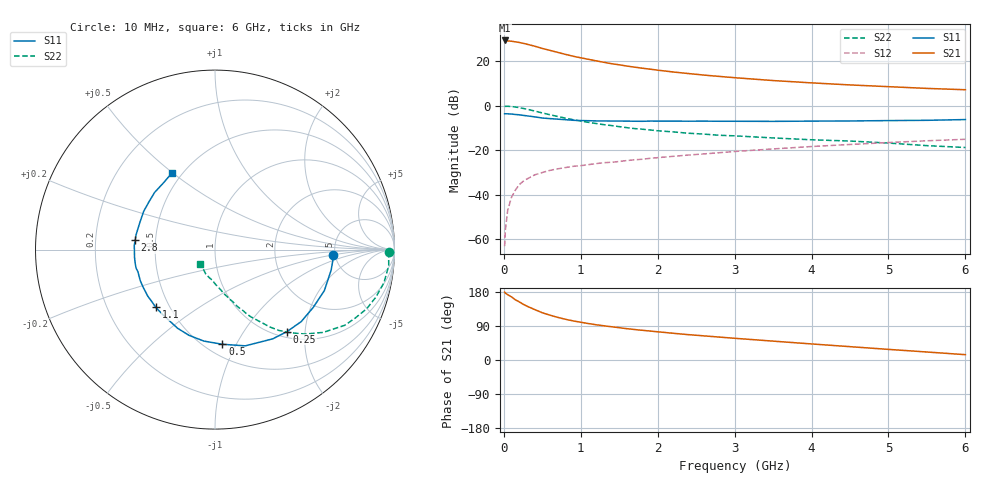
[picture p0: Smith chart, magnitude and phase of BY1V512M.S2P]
! SIEMENS Small Signal Semiconductors
! BFY420
! Si NPN RF SIEGET Grounded Emitter Transistor in MICRO-X
! VCE = 1.5 V  IC = 12 mA
! Common Emitter S-Parameters:  October  1996
# GHz  S  MA  R  50
!  f  S11  S21  S12  S22
! GHz  MAG  ANG  MAG  ANG  MAG  ANG  MAG  ANG
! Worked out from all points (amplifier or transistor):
!   36 points, 10 MHz to 6 GHz, reference 50 ohm
!   highest |S21| = 29.3 dB at 10 MHz (marker M1)
!   |S21| within 3 dB of that: start of sweep to 442.8 MHz
!   unconditionally stable (mu >= 1): 2.306 GHz to end of sweep
!   at 250 MHz: K = 0.22, MSG = 31.0 dB, |S12| = -34.0 dB
!   at 1.4 GHz: K = 0.81, MSG = 22.1 dB, |S12| = -25.4 dB
!   at 6 GHz: K = 1.10, MAG = 9.2 dB, |S12| = -15.1 dB
!   S11 on the Smith chart (normalised r, x): 10 MHz: 4.82, -0.47; 250 MHz: 1.11, -1.61; 500 MHz: 0.60, -0.88; 1.1 GHz: 0.42, -0.34; 2.8 GHz: 0.38, +0.05; 6 GHz: 0.44, +0.49
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0.01  0.6591 -2.4  29.24 179.1  0.0007 86.8  0.9713 -0.8
0.02  0.6601 -4.5  29.21 176.4  0.0016 86.1  0.968 -1.9
0.05  0.6572 -10.0  28.47 172.4  0.0045 81.5  0.9722 -5.3
0.1  0.6507 -20.6  28.13 166.5  0.0088 81.4  0.9592 -11.1
0.15  0.6351 -30.4  27.21 158.9  0.0127 75.8  0.9349 -16.4
0.2  0.6258 -39.9  26.41 153.5  0.0168 72.6  0.9073 -21.3
0.25  0.608 -48.7  25.27 147.3  0.02 68.2  0.8703 -25.9
0.3  0.5922 -57.1  24.07 142.1  0.0226 65.6  0.8375 -30.2
0.4  0.5622 -72.5  21.77 133.2  0.0279 61.0  0.7593 -37.4
0.5  0.5292 -85.5  19.35 124.7  0.0316 57.2  0.6886 -43.1
0.6  0.5134 -97.0  17.47 118.3  0.0353 54.2  0.6266 -47.7
0.8  0.4854 -115.4  14.24 107.5  0.0408 50.5  0.5264 -54.8
0.9  0.4709 -122.6  12.94 103.2  0.0435 50.1  0.4853 -57.2
1.1  0.4608 -135.7  11.03 96.1  0.0475 49.8  0.4235 -62.0
1.3  0.4556 -145.2  9.449 90.3  0.0525 49.1  0.3754 -65.2
1.6  0.4509 -157.6  7.766 82.6  0.0587 48.9  0.3214 -70.0
2.2  0.4505 -174.4  5.727 70.6  0.073 48.0  0.2583 -77.3
2.8  0.4477 173.3  4.552 60.5  0.0879 46.0  0.2168 -83.6
3.5  0.4451 160.3  3.675 49.8  0.107 42.4  0.189 -90.3
4.5  0.4543 144.0  2.931 35.2  0.1347 35.3  0.1609 -100.8
5.5  0.47 127.5  2.449 21.1  0.1631 26.8  0.1268 -120.5
6  0.4886 119.7  2.286 14.1  0.1762 22.1  0.1152 -134.6
